(* Logix 5000 Rung export; software revision 16.04 *)

MODULES
   Local : vendor None type None code None
   MNETC : vendor None type None code None
END_MODULES

TYPE MNETCEVENTCMD_SINGLE :   // Data structure to use for Event message generation.
STRUCT
   IP0 : INT;   // First digit of IP address
   IP1 : INT;   // Second digit of IP address
   IP2 : INT;   // Third digit of IP address
   IP3 : INT;   // Last digit of IP address
   ServPort : INT;   // TCP Service Port number (0-65535), 502 for MBAP, 2000 for MNET
   Node : INT;   // Modbus slave node address (0 to 247)
   DBAddress : INT;   // Module internal database to use with message
   Count : INT;   // Register or data point count
   Swap : INT;   // Swap code to use with functions 3 and 4
   Function : INT;   // Modbus function code for message
   Address : INT;   // Address to interface with in device
END_STRUCT
END_TYPE

TYPE MNETCSERVERSTATS :
STRUCT
   Requests : INT;   // Total number of request sent
   Responses : INT;   // Total number of responses received
   ErrSent : INT;   // Total number of errors sent
   ErrRec : INT;   // Total number of errors received
END_STRUCT
END_TYPE

TYPE MNETCEVENTCMD_SEQSTAT :   // Event Command Sequence Status for one client
STRUCT
   Trigger : BOOL;   // Triggers event sequence command
   ClientID : INT;   // Selects ClientID
   Client : MNETCEVENTCMD_SEQSTAT_CLIENT[30];   // Error Status Event
END_STRUCT
END_TYPE

TYPE MNETCCMDCONTROL :   // MVI56E-MNETC Command Control
STRUCT
   ClientID : INT;   // Block5000 Client Identification by Index number 0 to 29
   CMDqty : INT;   // Block5000 command quantity
   CmdIndex : INT[16];   // Contains index in the command list for the 1st command to be entered into Command queue
   WriteCmdBits : INT[30];   // Command Bit control ClientID(0 to 29)
END_STRUCT
END_TYPE

TYPE MNETCEVENTCMD :   // Event command data structure
STRUCT
   Trigger : BOOL;   // Triggers event command
   ClientID : INT;   // Client ID for event command
   Cmd : MNETCEVENTCMD_SINGLE[30];   // Event command list
END_STRUCT
END_TYPE

TYPE MNETCIPADDRESS :   // Data structure to get and set the IP address of the module.
STRUCT
   IPGetTrigger : BOOL;   // Gets IP address.
   IPReceived : INT[4];   // IP address received.
   IPSetTrigger : BOOL;   // Sets IP address
   IPRequested : INT[4];   // IP address set.
END_STRUCT
END_TYPE

TYPE MNETCMODULEDEF :   // This defines the whole module which includes all tags used in the program
STRUCT
   DATA : MNETCDATA;   // Data read from module
   CONTROL : MNETCCONTROL;   // Client ,Server Status and blocks status
   STATUS : MNETCSTATUS;   // MNETC Module control
   UTIL : MNETCUTIL;   // Block statistics
END_STRUCT
END_TYPE

TYPE MNETCBLOCKSTATS :   // This object is used to store the block transfer statistics for the MVI56E-MNETC module.
STRUCT
   Read : INT;   // Total number of read block transfers
   Write : INT;   // Total number of write block transfers
   Parse : INT;   // Total number of blocks parsed
   Event : INT;   // Total number of event blocks received
   Cmd : INT;   // Total number of command blocks received
   Err : INT;   // Total number of block transfer errors
END_STRUCT
END_TYPE

TYPE MNETCINITOUTDATA :   // Used to bring the Module into a known state after a restart operation.
STRUCT
   InitOutBlkIDLim : INT;   // Block Index Limit for ReadData size of the array
END_STRUCT
END_TYPE

TYPE MNETCUTIL :   // Values used by program for data transfer operation between the module and the processor.
STRUCT
   LastRead : INT;   // Index of last read block
   LastWrite : INT;   // Index of last write block
   BlockIndex : INT;   // Computed block offset for data table
   StatusIndex : INT;   // Computed block offset for status data
   ReadDataSizeGet : INT;   // Gets ReadData Array Length.
   WriteDataSizeGet : INT;   // Gets WriteData Array Length.
   ReadDataBlkCount : INT;   // Holds the value of the Block Counts of the Read Data Array.
   WriteDataBlkCount : INT;   // Holds the value of the Block Counts of the Write Data Array.
   RBTSremainder : INT;   // Holds remainder calculation value from the read array.
   WBTSremainder : INT;   // Holds remainder calculation value from the write array.
   PassThru : MNETCPASSTHRU;
   IPsetPending : BOOL;   // Allows Setting module IP address
   IPgetPending : BOOL;   // Allows Getting module IP address
   InitOutputData : MNETCINITOUTDATA;
   FaultCode : INT;   // Fault Code value
   CheckInitialization : BOOL;   // Check Initialization trigger
   StatusSeqIndex : INT;   // Computed block offset for status data
END_STRUCT
END_TYPE

TYPE MNETCCONTROL :   // Values used by program for data transfer operation between the module and the processor.
STRUCT
   BootTimer : TIMER;   // Timer used to clear both cold and warm boot requests
   ColdBoot : BOOL;   // Hardware reset of the Module
   WarmBoot : BOOL;   // Configuration data reset in the Module.
   ResetStatus : BOOL;   // Resets module status
   CmdID : INT;   // Command ID from 1 to 16
   CmdControl : MNETCCMDCONTROL;   // Holds Command Control statistics
   CmdControlPending : BOOL;   // Halts rung until Module is ready.
   CmdControlTrigger : BOOL;   // Command Control Trigger
   IPAddress : MNETCIPADDRESS;   // Getting and Setting IP address to and from Module
   EventCmd : MNETCEVENTCMD;   // Holds Event Command configuration
   EventSeqCmd : MNETCEVENTCMD_SEQ;   // Event Sequence Commands
END_STRUCT
END_TYPE

TYPE MNETCCMDCLIENTSEQ_PENDING :   // Event sequence event cmd pending status
STRUCT
   Trigger : BOOL;   // Triggers event sequence cmd pending status
   Client0_QueueCount : SINT;   // Command queue count for client 0
   Client0_WaitingMsgs : SINT;   // Event sequence messages waiting for client 0
   Client1_QueueCount : SINT;   // Command queue count for client 1
   Client1_WaitingMsgs : SINT;   // Event sequence messages waiting for client 1
   Client2_QueueCount : SINT;   // Command queue count for client 2
   Client2_WaitingMsgs : SINT;   // Event sequence messages waiting for client 2
   Client3_QueueCount : SINT;   // Command queue count for client 3
   Client3_WaitingMsgs : SINT;   // Event sequence messages waiting for client 3
   Client4_QueueCount : SINT;   // Command queue count for client 4
   Client4_WaitingMsgs : SINT;   // Event sequence messages waiting for client 4
   Client5_QueueCount : SINT;   // Command queue count for client 5
   Client5_WaitingMsgs : SINT;   // Event sequence messages waiting for client 5
   Client6_QueueCount : SINT;   // Command queue count for client 6
   Client6_WaitingMsgs : SINT;   // Event sequence messages waiting for client 6
   Client7_QueueCount : SINT;   // Command queue count for client 7
   Client7_WaitingMsgs : SINT;   // Event sequence messages waiting for client 7
   Client8_QueueCount : SINT;   // Command queue count for client 8
   Client8_WaitingMsgs : SINT;   // Event sequence messages waiting for client 8
   Client9_QueueCount : SINT;   // Command queue count for client 9
   Client9_WaitingMsgs : SINT;   // Event sequence messages waiting for client 9
   Client10_QueueCount : SINT;   // Command queue count for client 10
   Client10_WaitingMsgs : SINT;   // Event sequence messages waiting for client 10
   Client11_QueueCount : SINT;   // Command queue count for client 11
   Client11_WaitingMsgs : SINT;   // Event sequence messages waiting for client 11
   Client12_QueueCount : SINT;   // Command queue count for client 12
   Client12_WaitingMsgs : SINT;   // Event sequence messages waiting for client 12
   Client13_QueueCount : SINT;   // Command queue count for client 13
   Client13_WaitingMsgs : SINT;   // Event sequence messages waiting for client 13
   Client14_QueueCount : SINT;   // Command queue count for client 14
   Client14_WaitingMsgs : SINT;   // Event sequence messages waiting for client 14
   Client15_QueueCount : SINT;   // Command queue count for client 15
   Client15_WaitingMsgs : SINT;   // Event sequence messages waiting for client 15
   Client16_QueueCount : SINT;   // Command queue count for client 16
   Client16_WaitingMsgs : SINT;   // Event sequence messages waiting for client 16
   Client17_QueueCount : SINT;   // Command queue count for client 17
   Client17_WaitingMsgs : SINT;   // Event sequence messages waiting for client 17
   Client18_QueueCount : SINT;   // Command queue count for client 18
   Client18_WaitingMsgs : SINT;   // Event sequence messages waiting for client 18
   Client19_QueueCount : SINT;   // Command queue count for client 19
   Client19_WaitingMsgs : SINT;   // Event sequence messages waiting for client 19
   Client20_QueueCount : SINT;   // Command queue count for client 20
   Client20_WaitingMsgs : SINT;   // Event sequence messages waiting for client 20
   Client21_QueueCount : SINT;   // Command count for client 21
   Client21_WaitingMsgs : SINT;   // Event sequence messages waiting for client 21
   Client22_QueueCount : SINT;   // Command queue count for client 22
   Client22_WaitingMsgs : SINT;   // Event sequence messages waiting for client 22
   Client23_QueueCount : SINT;   // Command queue count for client 23
   Client23_WaitingMsgs : SINT;   // Event sequence messages waiting for client 23
   Client24_QueueCount : SINT;   // Command queue count for client 24
   Client24_WaitingMsgs : SINT;   // Event sequence messages waiting for client 24
   Client25_QueueCount : SINT;   // Command queue count for client 25
   Client25_WaitingMsgs : SINT;   // Event sequence messages waiting for client 25
   Client26_QueueCount : SINT;   // Command queue count for client 26
   Client26_WaitingMsgs : SINT;   // Event sequence messages waiting for client 26
   Client27_QueueCount : SINT;   // Command queue count for client 27
   Client27_WaitingMsgs : SINT;   // Event sequence messages waiting for client 27
   Client28_QueueCount : SINT;   // Command queue count for client 28
   Client28_WaitingMsgs : SINT;   // Event sequence message waiting for client 28
   Client29_QueueCount : SINT;   // Command queue count for client 29
   Client29_WaitingMsgs : SINT;   // Event sequence messages waiting for client 29
END_STRUCT
END_TYPE

TYPE MNETCEVENTCMD_SEQ :   // Data structure to use for each event command with status tracking by sequence number (blocks 4000 to 4029).
STRUCT
   Trigger : BOOL;   // Trigger Event Sequence Command
   ClientID : INT;   // Client ID for event sequence command (0-29)
   IP0 : INT;   // First digit of IP address
   IP1 : INT;   // Second digit of IP address
   IP2 : INT;   // Third digit of IP address
   IP3 : INT;   // Last digit of IP address
   ServPort : INT;   // TCP Service Port number (0-65535), 502 for MBAP, 2000 for MNET
   Node : INT;   // Modbus slave node address (0 to 247)
   DBAddress : INT;   // Module internal database to use with message
   Count : INT;   // Register or data point count
   Swap : INT;   // Swap code to use with functions 3 and 4
   Function : INT;   // Modbus function code for message
   Address : INT;   // Address to interface within device
   Sequence : INT;   // Unique sequence number to keep track of status code
END_STRUCT
END_TYPE

TYPE MNETCDATA :   // Contains Read Data (data read from the module to the processor) and Write Data (data written from the processor to the module)
STRUCT
   ReadData : INT[600];   // Data read from module. Set array equal to the size set in the Configuration file.
   WriteData : INT[600];   // Data to write to module. Set array equal to the size set in the Configuration file.
END_STRUCT
END_TYPE

TYPE MNETCSERVERS :   // This object is used to store the Server statistics for an MVI56E-MNETC port.
STRUCT
   MNET : MNETCSERVERSTATS;   // Server status for TCP port 2000
   MBAP : MNETCSERVERSTATS;   // Server status for TCP port 502
END_STRUCT
END_TYPE

TYPE MNETCEVENTCMD_SEQSTAT_SEQ_ERR :   // Mnet event status of sequence event commands
STRUCT
   Sequence : INT;   // Sequence Number
   Error : INT;   // Error Code
END_STRUCT
END_TYPE

TYPE MNETCEVENTCMD_SEQSTAT_CLIENT :   // Event Command Sequence Status for one client
STRUCT
   Count : INT;   // Number of event commands received
   Cmd : MNETCEVENTCMD_SEQSTAT_SEQ_ERR[15];   // Error Status Event
END_STRUCT
END_TYPE

TYPE MNETCPASSTHRU :
STRUCT
   MBControl1 : CONTROL;   // Modbus pass thru message control
   MBControl2 : CONTROL;   // Modbus pass thru message control
   Mbdouble : DINT;   // Modbus double int tag
   MBMsg : SINT[500];   // Message array
   MBMsgLen : INT;   // Message length
   MBOffset : INT;   // Start offset in the message
   MBOffsetBit : INT;   // Offset bit in the message
   MBScratch : INT[3];   // Temporary used ints
   MBboolLength : DINT;   // Holds Word size that will accommodate Coil Qty.
   MBSpecial : INT[4];   // Holds Special Function 99 data.
   And_Mask : INT;   // Function 22 "AND" Mask
   Or_Mask : INT;   // Function 22 "OR" Mask
END_STRUCT
END_TYPE

TYPE MNETCCLIENTSTATS :   // This object is used to store the port statistics for an MVI56E-MNETC port.
STRUCT
   CmdReq : INT;   // Total number of command list requests sent
   CmdResp : INT;   // Total number of command list responses received
   CmdErr : INT;   // Total number of command list errors
   Requests : INT;   // Total number of requests for port
   Responses : INT;   // Total number of responses for port
   ErrSent : INT;   // Total number of errors sent
   ErrRec : INT;   // Total number of errors received
   CfgErrWord : INT;   // Configuration Error Word
   CurErr : INT;   // Current Error code
   LastErr : INT;   // Last recorded error code
END_STRUCT
END_TYPE

TYPE MNETCSTATUS :   // This status data is returned on each read block and can be used to detect proper module operation.
STRUCT
   PassCnt : INT;   // Program cycle counter
   ProductVersion : INT;   // This is used to pass the product version to the processor
   ProductCode : INT[2];   // This is used to pass the product Code to the processor
   BlockStats : MNETCBLOCKSTATS;   // Block transfer statistics
   CmdBits : INT[30];   // Commands bits array to be used for 30 clients
   ClientStatsTrigger : BOOL;   // Get Client Status
   ClientID : INT;   // Client ID to get Status From
   ClientStatus : MNETCCLIENTSTATS[30];   // Client status data
   CmdErrorList : INT[16];   // Command Error List
   EventSeqCmdPending : MNETCCMDCLIENTSEQ_PENDING;   // Stores information on the number of seq events pending in the module
   EventSeqCmd : MNETCEVENTCMD_SEQSTAT;   // Event seq event commands pending
   EventSeqReady : DINT;   // Bit mapped for Status data (bit=1 data ready, bit = 0 no event data)
   ServerStatsTrigger : BOOL;   // Get Server Status
   ServerStatus : MNETCSERVERS;   // Server status data
END_STRUCT
END_TYPE

ADD_ON_INSTRUCTION AOI56MNETC   (* revision 1.10, vendor ProSoft Technology Inc., ExecutePrescan *)
// Add-On for  MVI56E-MNETC modules with firmware version 3.01 and newer.
// Revision note:
// v1.10 -  Enables all commands as a default by setting all WriteCmdBits to 1.
VAR_IN_OUT
   Connection_Input : INT[250]; {required}   // Input parameters.
   Connection_Output : INT[248]; {required}   // Output parameters.
   MNETC : MNETCMODULEDEF; {required}
END_VAR
VAR
   MJFAULTS : DINT[12];
END_VAR

ROUTINE Logic   (* ladder *)
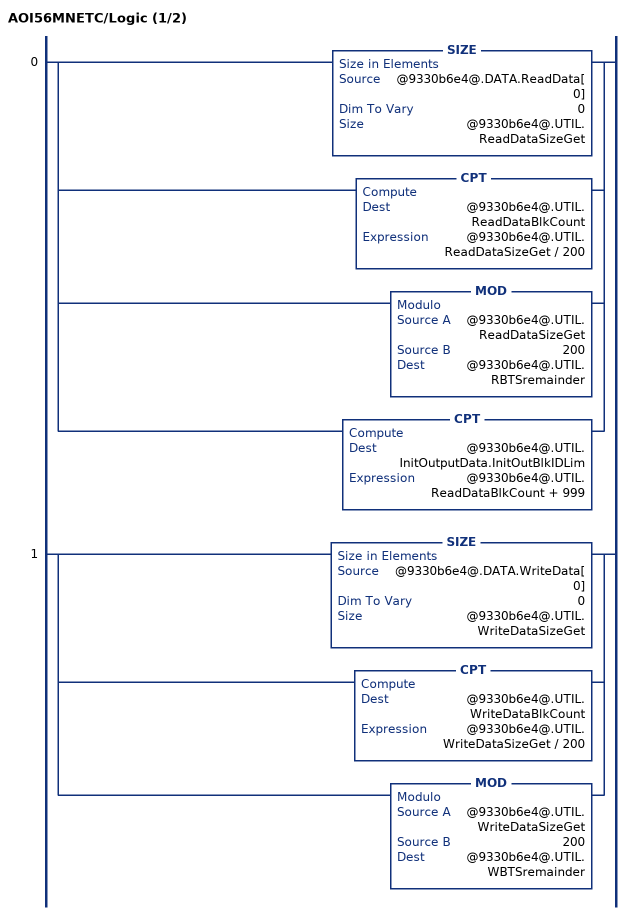
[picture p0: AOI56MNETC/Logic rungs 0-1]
   0: [SIZE(@9330b6e4@.DATA.ReadData[0],0,@9330b6e4@.UTIL.ReadDataSizeGet) ,CPT(@9330b6e4@.UTIL.ReadDataBlkCount,@9330b6e4@.UTIL.ReadDataSizeGet / 200) ,MOD(@9330b6e4@.UTIL.ReadDataSizeGet,200,@9330b6e4@.UTIL.RBTSremainder) ,CPT(@9330b6e4@.UTIL.InitOutputData.InitOutBlkIDLim,@9330b6e4@.UTIL.ReadDataBlkCount + 999) ];
   1: [SIZE(@9330b6e4@.DATA.WriteData[0],0,@9330b6e4@.UTIL.WriteDataSizeGet) ,CPT(@9330b6e4@.UTIL.WriteDataBlkCount,@9330b6e4@.UTIL.WriteDataSizeGet / 200) ,MOD(@9330b6e4@.UTIL.WriteDataSizeGet,200,@9330b6e4@.UTIL.WBTSremainder) ];
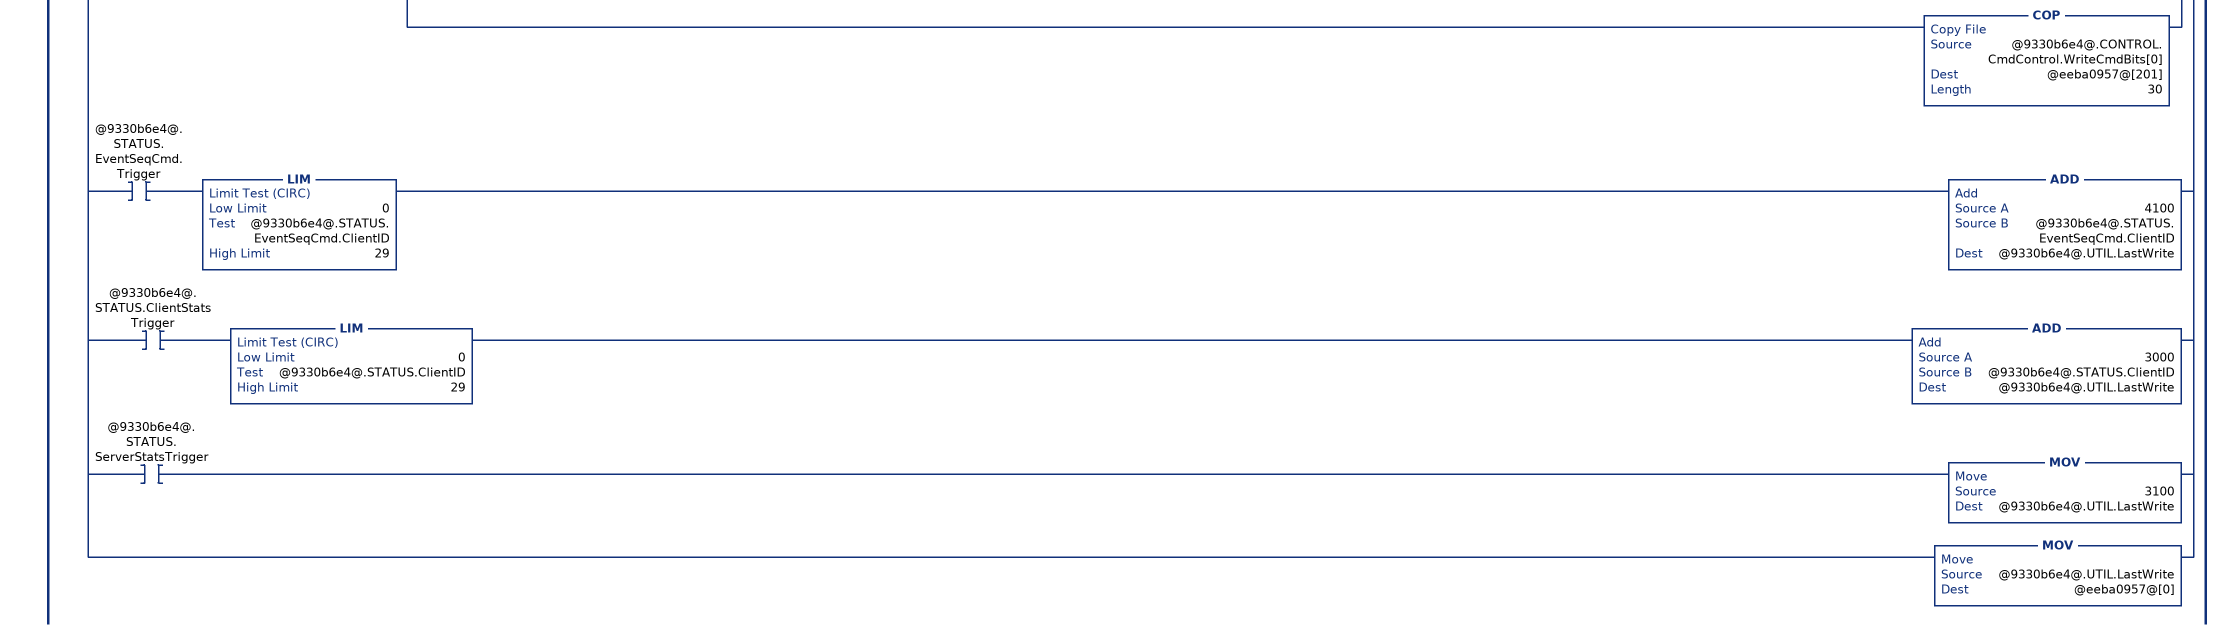
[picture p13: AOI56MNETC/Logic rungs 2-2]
   2: NEQ(@162e95de@[249],@9330b6e4@.UTIL.LastRead)[MOV(@162e95de@[249],@9330b6e4@.UTIL.LastRead) ,GRT(@9330b6e4@.UTIL.FaultCode,0) OTL(@9330b6e4@.UTIL.CheckInitialization) ,EQU(@9330b6e4@.UTIL.FaultCode,0) NEQ(@9330b6e4@.UTIL.LastRead,0) OTU(@9330b6e4@.UTIL.CheckInitialization) ,EQU(@9330b6e4@.UTIL.FaultCode,0) [EQU(-1,@9330b6e4@.UTIL.LastRead) ,EQU(0,@9330b6e4@.UTIL.LastRead) ] XIO(@9330b6e4@.UTIL.CheckInitialization) [[EQU(@9330b6e4@.STATUS.ProductCode[1],13637) GEQ(@9330b6e4@.STATUS.ProductVersion,204) ,EQU(@9330b6e4@.STATUS.ProductCode[1],13635) GEQ(@9330b6e4@.STATUS.ProductVersion,113) ] [GEQ(@9330b6e4@.UTIL.ReadDataSizeGet,200) COP(@162e95de@[2],@9330b6e4@.DATA.ReadData[0],200) ,LES(@9330b6e4@.UTIL.ReadDataSizeGet,200) COP(@162e95de@[2],@9330b6e4@.DATA.ReadData[0],@9330b6e4@.UTIL.RBTSremainder) ] ,COP(@162e95de@[202],@9330b6e4@.STATUS.PassCnt,1) ,COP(@162e95de@[203],@9330b6e4@.STATUS.BlockStats.Read,6) ,COP(@162e95de@[209],@9330b6e4@.STATUS.CmdBits[0],30) ,COP(@162e95de@[239],@9330b6e4@.STATUS.ProductCode[0],2) ,COP(@162e95de@[241],@9330b6e4@.STATUS.ProductVersion,1) ,COP(@162e95de@[242],@9330b6e4@.STATUS.EventSeqReady,1) ] ,GEQ(@9330b6e4@.UTIL.LastRead,1) [LEQ(@9330b6e4@.UTIL.LastRead,@9330b6e4@.UTIL.ReadDataBlkCount) [CPT(@9330b6e4@.UTIL.BlockIndex,(@9330b6e4@.UTIL.LastRead-1)*200) ,COP(@162e95de@[2],@9330b6e4@.DATA.ReadData[@9330b6e4@.UTIL.BlockIndex],200) ,COP(@162e95de@[202],@9330b6e4@.STATUS.PassCnt,1) ,COP(@162e95de@[203],@9330b6e4@.STATUS.BlockStats.Read,6) ,COP(@162e95de@[209],@9330b6e4@.STATUS.CmdBits[0],30) ,COP(@162e95de@[239],@9330b6e4@.STATUS.ProductCode[0],2) ,COP(@162e95de@[241],@9330b6e4@.STATUS.ProductVersion,1) ,COP(@162e95de@[242],@9330b6e4@.STATUS.EventSeqReady,1) ] ,CMP(@9330b6e4@.UTIL.LastRead - @9330b6e4@.UTIL.ReadDataBlkCount = 1) GRT(@9330b6e4@.UTIL.RBTSremainder,0) [CPT(@9330b6e4@.UTIL.BlockIndex,(@9330b6e4@.UTIL.LastRead - 1) * 200) ,COP(@162e95de@[2],@9330b6e4@.DATA.ReadData[@9330b6e4@.UTIL.BlockIndex],@9330b6e4@.UTIL.RBTSremainder) ,COP(@162e95de@[202],@9330b6e4@.STATUS.PassCnt,1) ,COP(@162e95de@[203],@9330b6e4@.STATUS.BlockStats.Read,6) ,COP(@162e95de@[209],@9330b6e4@.STATUS.CmdBits[0],30) ,COP(@162e95de@[239],@9330b6e4@.STATUS.ProductCode[0],2) ,COP(@162e95de@[241],@9330b6e4@.STATUS.ProductVersion,1) ,COP(@162e95de@[242],@9330b6e4@.STATUS.EventSeqReady,1) ] ] ,LIM(9956,@9330b6e4@.UTIL.LastRead,9996) [EQU(9996,@9330b6e4@.UTIL.LastRead) [MOV(@162e95de@[2],@9330b6e4@.UTIL.PassThru.MBMsgLen) ,COP(@162e95de@[4],@9330b6e4@.UTIL.PassThru.MBMsg[0],@9330b6e4@.UTIL.PassThru.MBMsgLen) ] ,LIM(9956,@9330b6e4@.UTIL.LastRead,9957) [MOV(@162e95de@[3],@9330b6e4@.UTIL.PassThru.MBOffset) ,LES(@9330b6e4@.UTIL.PassThru.MBOffset,@9330b6e4@.UTIL.WriteDataSizeGet) COP(@162e95de@[4],@9330b6e4@.DATA.WriteData[@9330b6e4@.UTIL.PassThru.MBOffset],@162e95de@[2]) ] ,EQU(9958,@9330b6e4@.UTIL.LastRead) [MOV(@162e95de@[3],@9330b6e4@.UTIL.PassThru.MBOffsetBit) ,MOV(@162e95de@[4],@9330b6e4@.UTIL.PassThru.MBScratch[2]) ,DIV(@9330b6e4@.UTIL.PassThru.MBOffsetBit,16,@9330b6e4@.UTIL.PassThru.MBOffset) ,MOD(@9330b6e4@.UTIL.PassThru.MBOffsetBit,16,@9330b6e4@.UTIL.PassThru.MBOffsetBit) ,XPY(2,@9330b6e4@.UTIL.PassThru.MBOffsetBit,@9330b6e4@.UTIL.PassThru.mbdouble) ,MVM(@9330b6e4@.UTIL.PassThru.mbdouble,16#0000_ffff,@9330b6e4@.UTIL.PassThru.MBOffsetBit) ,GEQ(@9330b6e4@.UTIL.PassThru.MBOffset,0) LES(@9330b6e4@.UTIL.PassThru.MBOffset,@9330b6e4@.UTIL.WriteDataSizeGet) LEQ(@9330b6e4@.UTIL.PassThru.MBOffset,2048) [NEQ(@9330b6e4@.UTIL.PassThru.MBScratch[2],0) OR(@9330b6e4@.UTIL.PassThru.MBOffsetBit,@9330b6e4@.DATA.WriteData[@9330b6e4@.UTIL.PassThru.MBOffset],@9330b6e4@.DATA.WriteData[@9330b6e4@.UTIL.PassThru.MBOffset]) ,EQU(@9330b6e4@.UTIL.PassThru.MBScratch[2],0) [NOT(@9330b6e4@.UTIL.PassThru.MBOffsetBit,@9330b6e4@.UTIL.PassThru.MBOffsetBit) ,AND(@9330b6e4@.UTIL.PassThru.MBOffsetBit,@9330b6e4@.DATA.WriteData[@9330b6e4@.UTIL.PassThru.MBOffset],@9330b6e4@.DATA.WriteData[@9330b6e4@.UTIL.PassThru.MBOffset]) ] ] ] ,EQU(9959,@9330b6e4@.UTIL.LastRead) [[MOV(@162e95de@[3],@9330b6e4@.UTIL.PassThru.MBOffset) ,MOV(@162e95de@[2],@9330b6e4@.UTIL.PassThru.MBControl1.LEN) ,MOV(@162e95de@[2],@9330b6e4@.UTIL.PassThru.MBControl2.LEN) ,CPT(@9330b6e4@.UTIL.PassThru.MBboolLength,@9330b6e4@.UTIL.PassThru.MBOffset+@9330b6e4@.UTIL.PassThru.MBControl1.LEN) ] ,LEQ(@9330b6e4@.UTIL.PassThru.MBboolLength,@9330b6e4@.UTIL.WriteDataSizeGet) [FAL(@9330b6e4@.UTIL.PassThru.MBControl1,?,?,ALL,@9330b6e4@.DATA.WriteData[@9330b6e4@.UTIL.PassThru.MBOffset+@9330b6e4@.UTIL.PassThru.MBControl1.POS],@9330b6e4@.DATA.WriteData[@9330b6e4@.UTIL.PassThru.MBOffset+@9330b6e4@.UTIL.PassThru.MBControl1.POS] AND(NOT @162e95de@[54+@9330b6e4@.UTIL.PassThru.MBControl1.POS])) ,FAL(@9330b6e4@.UTIL.PassThru.MBControl2,?,?,ALL,@9330b6e4@.DATA.WriteData[@9330b6e4@.UTIL.PassThru.MBOffset+@9330b6e4@.UTIL.PassThru.MBControl2.POS],@9330b6e4@.DATA.WriteData[@9330b6e4@.UTIL.PassThru.MBOffset+@9330b6e4@.UTIL.PassThru.MBControl2.POS] OR(@162e95de@[54+@9330b6e4@.UTIL.PassThru.MBControl2.POS] AND @162e95de@[4+@9330b6e4@.UTIL.PassThru.MBControl2.POS])) ,RES(@9330b6e4@.UTIL.PassThru.MBControl1) ,RES(@9330b6e4@.UTIL.PassThru.MBControl2) ] ] ,EQU(@9330b6e4@.UTIL.LastRead,9960) LIM(0,@162e95de@[3],@9330b6e4@.UTIL.WriteDataSizeGet) [MOV(@162e95de@[3],@9330b6e4@.UTIL.PassThru.MBOffset) ,MOV(@162e95de@[4],@9330b6e4@.UTIL.PassThru.And_Mask) ,MOV(@162e95de@[5],@9330b6e4@.UTIL.PassThru.Or_Mask) ,CPT(@9330b6e4@.DATA.WriteData[@9330b6e4@.UTIL.PassThru.MBOffset],(@9330b6e4@.DATA.WriteData[@9330b6e4@.UTIL.PassThru.MBOffset] AND @9330b6e4@.UTIL.PassThru.And_Mask)OR(@9330b6e4@.UTIL.PassThru.Or_Mask AND (NOT(@9330b6e4@.UTIL.PassThru.And_Mask)))) ] ,EQU(@9330b6e4@.UTIL.LastRead,9961) LIM(0,@162e95de@[3],@9330b6e4@.UTIL.WriteDataSizeGet) [MOV(@162e95de@[3],@9330b6e4@.UTIL.PassThru.MBOffset) ,MOV(@162e95de@[2],@9330b6e4@.UTIL.PassThru.MBMsgLen) ,COP(@162e95de@[4],@9330b6e4@.DATA.WriteData[@9330b6e4@.UTIL.PassThru.MBOffset],@9330b6e4@.UTIL.PassThru.MBMsgLen) ] ,EQU(9970,@9330b6e4@.UTIL.LastRead) COP(@eeba0957@[0],@9330b6e4@.UTIL.PassThru.MBSpecial[0],4) ] ,LIM(3000,@9330b6e4@.UTIL.LastRead,3029) [CPT(@9330b6e4@.UTIL.StatusIndex,@9330b6e4@.UTIL.LastRead-3000) ,COP(@162e95de@[3],@9330b6e4@.STATUS.ClientStatus[@9330b6e4@.UTIL.StatusIndex].CmdReq,10) ,COP(@162e95de@[13],@9330b6e4@.STATUS.CmdErrorList[0],16) ,OTU(@9330b6e4@.STATUS.ClientStatsTrigger) ] ,EQU(3100,@9330b6e4@.UTIL.LastRead) [[COP(@162e95de@[6],@9330b6e4@.STATUS.ServerStatus.MNET.Requests,4) ,COP(@162e95de@[16],@9330b6e4@.STATUS.ServerStatus.MBAP.Requests,4) ] ,OTU(@9330b6e4@.STATUS.ServerStatsTrigger) ] ,EQU(@9330b6e4@.UTIL.LastRead,9990) [COP(@162e95de@[2],@9330b6e4@.CONTROL.IPAddress.IPRequested[0],4) ,OTU(@9330b6e4@.UTIL.IPsetPending) ] ,EQU(@9330b6e4@.UTIL.LastRead,9991) [COP(@162e95de@[2],@9330b6e4@.CONTROL.IPAddress.IPReceived[0],4) ,OTU(@9330b6e4@.UTIL.IPgetPending) ] ,XIC(@9330b6e4@.CONTROL.CmdControlTrigger) LIM(5001,@9330b6e4@.UTIL.LastRead,5016) LIM(1,@162e95de@[2],16) OTU(@9330b6e4@.CONTROL.CmdControlTrigger) ,XIC(@9330b6e4@.CONTROL.EventCmd.Trigger) LIM(2000,@9330b6e4@.UTIL.LastRead,2029) EQU(@162e95de@[2],1) OTU(@9330b6e4@.CONTROL.EventCmd.Trigger) ,XIC(@9330b6e4@.CONTROL.EventSeqCmd.Trigger) LIM(4000,@9330b6e4@.UTIL.LastRead,4029) EQU(@162e95de@[2],1) OTU(@9330b6e4@.CONTROL.EventSeqCmd.Trigger) ,LIM(4100,@9330b6e4@.UTIL.LastRead,4129) [CPT(@9330b6e4@.UTIL.StatusSeqIndex,@9330b6e4@.UTIL.LastRead-4100) ,COP(@162e95de@[2],@9330b6e4@.STATUS.EventSeqCmd.Client[@9330b6e4@.UTIL.StatusSeqIndex].Count,1) ,COP(@162e95de@[3],@9330b6e4@.STATUS.EventSeqCmd.Client[@9330b6e4@.UTIL.StatusSeqIndex].Cmd[0],30) ,OTU(@9330b6e4@.STATUS.EventSeqCmd.Trigger) ] ,EQU(@9330b6e4@.UTIL.LastRead,4200) COP(@162e95de@[2],@9330b6e4@.STATUS.EventSeqCmdPending.Client0_QueueCount,60) ,MOV(@162e95de@[1],@9330b6e4@.UTIL.LastWrite) ,XIC(@9330b6e4@.CONTROL.WarmBoot) [MOV(9998,@9330b6e4@.UTIL.LastWrite) ,OTU(@9330b6e4@.CONTROL.WarmBoot) ] ,XIC(@9330b6e4@.CONTROL.ColdBoot) [MOV(9999,@9330b6e4@.UTIL.LastWrite) ,OTU(@9330b6e4@.CONTROL.ColdBoot) ] ,XIC(@9330b6e4@.CONTROL.ResetStatus) [MOV(9997,@9330b6e4@.UTIL.LastWrite) ,OTU(@9330b6e4@.CONTROL.ResetStatus) ] ,XIC(@9330b6e4@.CONTROL.IPAddress.IPSetTrigger) XIO(@9330b6e4@.UTIL.IPsetPending) [COP(@9330b6e4@.CONTROL.IPAddress.IPRequested[0],@eeba0957@[1],4) ,MOV(9990,@9330b6e4@.UTIL.LastWrite) ,OTU(@9330b6e4@.CONTROL.IPAddress.IPSetTrigger) ,OTL(@9330b6e4@.UTIL.IPsetPending) ] ,XIC(@9330b6e4@.CONTROL.IPAddress.IPGetTrigger) XIO(@9330b6e4@.UTIL.IPgetPending) [MOV(9991,@9330b6e4@.UTIL.LastWrite) ,OTU(@9330b6e4@.CONTROL.IPAddress.IPGetTrigger) ,OTL(@9330b6e4@.UTIL.IPgetPending) ] ,XIC(@9330b6e4@.CONTROL.CmdControlTrigger) LIM(1,@9330b6e4@.CONTROL.CmdID,16) [LIM(0,@9330b6e4@.CONTROL.CmdControl.ClientID,29) MOV(@9330b6e4@.CONTROL.CmdControl.ClientID,@eeba0957@[1]) ,COP(@9330b6e4@.CONTROL.CmdControl.CmdIndex[0],@eeba0957@[2],16) ,ADD(5000,@9330b6e4@.CONTROL.CmdID,@9330b6e4@.UTIL.LastWrite) ] ,XIC(@9330b6e4@.CONTROL.EventSeqCmd.Trigger) LIM(0,@9330b6e4@.CONTROL.EventSeqCmd.ClientID,29) [ADD(4000,@9330b6e4@.CONTROL.EventSeqCmd.ClientID,@9330b6e4@.UTIL.LastWrite) ,COP(@9330b6e4@.CONTROL.EventSeqCmd.IP0,@eeba0957@[1],12) ] ,XIC(@9330b6e4@.CONTROL.EventCmd.Trigger) LIM(0,@9330b6e4@.CONTROL.EventCmd.ClientID,29) [ADD(2000,@9330b6e4@.CONTROL.EventCmd.ClientID,@9330b6e4@.UTIL.LastWrite) ,COP(@9330b6e4@.CONTROL.EventCmd.Cmd[@9330b6e4@.CONTROL.EventCmd.ClientID].IP0,@eeba0957@[1],11) ] ,XIC(@9330b6e4@.STATUS.EventSeqCmdPending.Trigger) [MOV(4200,@9330b6e4@.UTIL.LastWrite) ,OTU(@9330b6e4@.STATUS.EventSeqCmdPending.Trigger) ] ,GEQ(@9330b6e4@.UTIL.LastWrite,1) [LEQ(@9330b6e4@.UTIL.LastWrite,@9330b6e4@.UTIL.WriteDataBlkCount) [CPT(@9330b6e4@.UTIL.BlockIndex,(@9330b6e4@.UTIL.LastWrite-1)*200) ,COP(@9330b6e4@.DATA.WriteData[@9330b6e4@.UTIL.BlockIndex],@eeba0957@[1],200) ,COP(@9330b6e4@.CONTROL.CmdControl.WriteCmdBits[0],@eeba0957@[201],30) ] ,CMP(@9330b6e4@.UTIL.LastWrite - @9330b6e4@.UTIL.WriteDataBlkCount = 1) GRT(@9330b6e4@.UTIL.WBTSremainder,0) [CPT(@9330b6e4@.UTIL.BlockIndex,(@9330b6e4@.UTIL.LastWrite - 1) * 200) ,COP(@9330b6e4@.DATA.WriteData[@9330b6e4@.UTIL.BlockIndex],@eeba0957@[1],@9330b6e4@.UTIL.WBTSremainder) ,COP(@9330b6e4@.CONTROL.CmdControl.WriteCmdBits[0],@eeba0957@[201],30) ] ] ,LIM(1000,@9330b6e4@.UTIL.LastWrite,1049) LEQ(@9330b6e4@.UTIL.LastWrite,@9330b6e4@.UTIL.InitOutputData.InitOutBlkIDLim) [CPT(@9330b6e4@.UTIL.BlockIndex,(@9330b6e4@.UTIL.LastWrite-1000)*200) ,COP(@9330b6e4@.DATA.ReadData[@9330b6e4@.UTIL.BlockIndex],@eeba0957@[1],200) ] ,[EQU(-1,@9330b6e4@.UTIL.LastWrite) ,EQU(0,@9330b6e4@.UTIL.LastWrite) ] [[EQU(@9330b6e4@.STATUS.ProductCode[1],13637) GEQ(@9330b6e4@.STATUS.ProductVersion,204) ,EQU(@9330b6e4@.STATUS.ProductCode[1],13635) GEQ(@9330b6e4@.STATUS.ProductVersion,113) ] [GEQ(@9330b6e4@.UTIL.WriteDataSizeGet,200) COP(@9330b6e4@.DATA.WriteData[0],@eeba0957@[1],200) ,LES(@9330b6e4@.UTIL.WriteDataSizeGet,200) COP(@9330b6e4@.DATA.WriteData[0],@eeba0957@[1],@9330b6e4@.UTIL.WBTSremainder) ] ,COP(@9330b6e4@.CONTROL.CmdControl.WriteCmdBits[0],@eeba0957@[201],30) ] ,XIC(@9330b6e4@.STATUS.EventSeqCmd.Trigger) LIM(0,@9330b6e4@.STATUS.EventSeqCmd.ClientID,29) ADD(4100,@9330b6e4@.STATUS.EventSeqCmd.ClientID,@9330b6e4@.UTIL.LastWrite) ,XIC(@9330b6e4@.STATUS.ClientStatsTrigger) LIM(0,@9330b6e4@.STATUS.ClientID,29) ADD(3000,@9330b6e4@.STATUS.ClientID,@9330b6e4@.UTIL.LastWrite) ,XIC(@9330b6e4@.STATUS.ServerStatsTrigger) MOV(3100,@9330b6e4@.UTIL.LastWrite) ,MOV(@9330b6e4@.UTIL.LastWrite,@eeba0957@[0]) ];
END_ROUTINE

ROUTINE Prescan   (* ladder *)
// Prescan
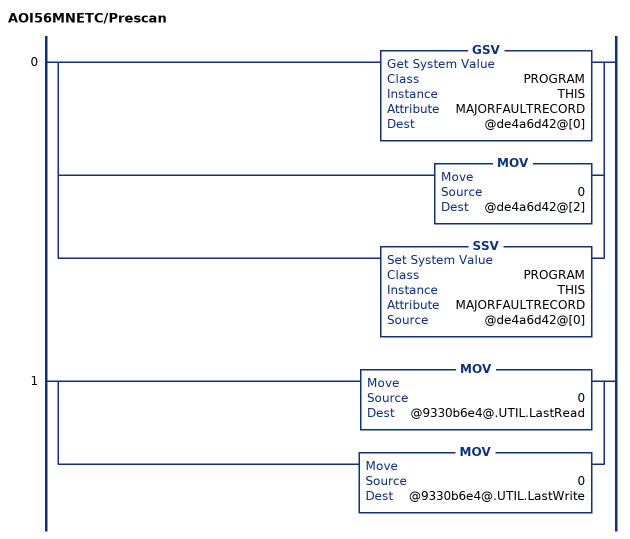
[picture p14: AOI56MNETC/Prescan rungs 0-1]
   0: [GSV(PROGRAM,THIS,MAJORFAULTRECORD,@de4a6d42@[0]) ,MOV(0,@de4a6d42@[2]) ,SSV(PROGRAM,THIS,MAJORFAULTRECORD,@de4a6d42@[0]) ];
   1: [MOV(0,@9330b6e4@.UTIL.LastRead) ,MOV(0,@9330b6e4@.UTIL.LastWrite) ];
END_ROUTINE
END_ADD_ON_INSTRUCTION

VAR_GLOBAL   (* controller tags *)
   AOI56MNETC : AOI56MNETC;
   Local:1:I : AB:1756_MODULE_INT_500Bytes:I:0;
   MNETC : MNETCMODULEDEF;
   Local:1:O : AB:1756_MODULE_INT_496Bytes:O:0;
END_VAR

PROGRAM MainProgram

ROUTINE MainRoutine   (* ladder *)
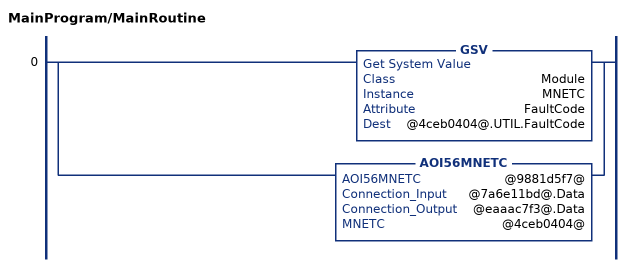
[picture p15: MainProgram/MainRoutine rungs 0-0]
   0: [GSV(Module,MNETC,FaultCode,@4ceb0404@.UTIL.FaultCode) ,AOI56MNETC(@9881d5f7@,@7a6e11bd@.Data,@eaaac7f3@.Data,@4ceb0404@) ];
END_ROUTINE
END_PROGRAM
